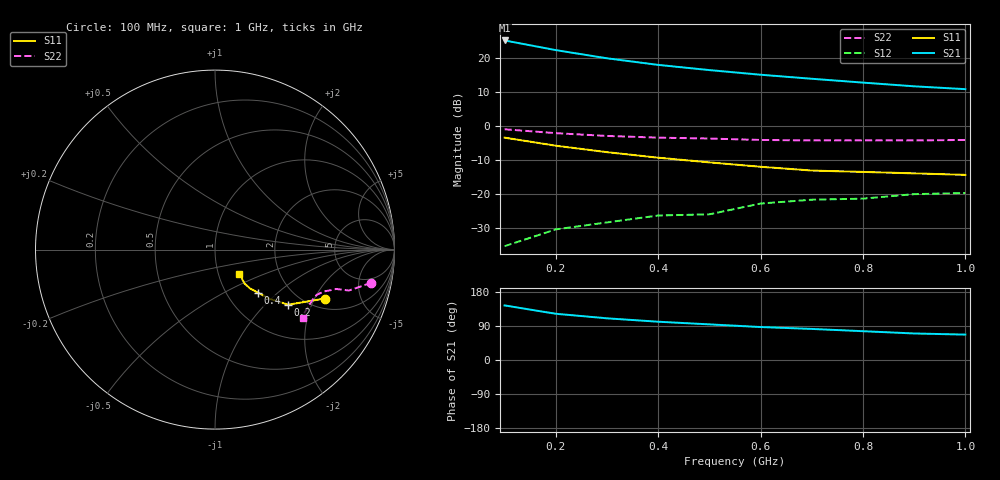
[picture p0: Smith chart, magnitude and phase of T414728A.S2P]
!AT-41472
!S-PARAMETERS at Vce=8V  Ic=10mA.  LAST UPDATED 07-21-92
# ghz s ma r 50
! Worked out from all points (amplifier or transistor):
!   10 points, 100 MHz to 1 GHz, reference 50 ohm
!   highest |S21| = 25.1 dB at 100 MHz (marker M1)
!   |S21| within 3 dB of that: start of sweep to 206.7 MHz
!   unconditionally stable (mu >= 1): 438.5 MHz to end of sweep
!   at 200 MHz: K = 0.72, MSG = 26.4 dB, |S12| = -30.5 dB
!   at 600 MHz: K = 1.01, MAG = 18.3 dB, |S12| = -22.9 dB
!   at 1 GHz: K = 1.11, MAG = 13.3 dB, |S12| = -19.7 dB
!   S11 on the Smith chart (normalised r, x): 100 MHz: 2.45, -2.43; 200 MHz: 1.66, -1.38; 400 MHz: 1.39, -0.76; 1 GHz: 1.26, -0.35
0.1  0.67 -24.0  18 144.0  0.017 71.0  0.89 -12.0
0.2  0.51 -37.0  12.98 122.0  0.03 71.0  0.78 -17.0
0.3  0.41 -42.0  9.84 110.0  0.038 72.0  0.71 -18.0
0.4  0.34 -45.0  7.87 101.0  0.048 71.0  0.67 -20.0
0.5  0.29 -48.0  6.6 94.0  0.05 71.0  0.65 -21.0
0.6  0.25 -49.0  5.64 87.0  0.072 71.0  0.62 -24.0
0.7  0.22 -47.0  4.92 82.0  0.082 69.0  0.61 -28.0
0.8  0.21 -45.0  4.32 76.0  0.085 67.0  0.61 -31.0
0.9  0.2 -45.0  3.81 70.0  0.099 64.0  0.61 -35.0
1  0.19 -45.0  3.46 67.0  0.103 64.0  0.62 -38.0
